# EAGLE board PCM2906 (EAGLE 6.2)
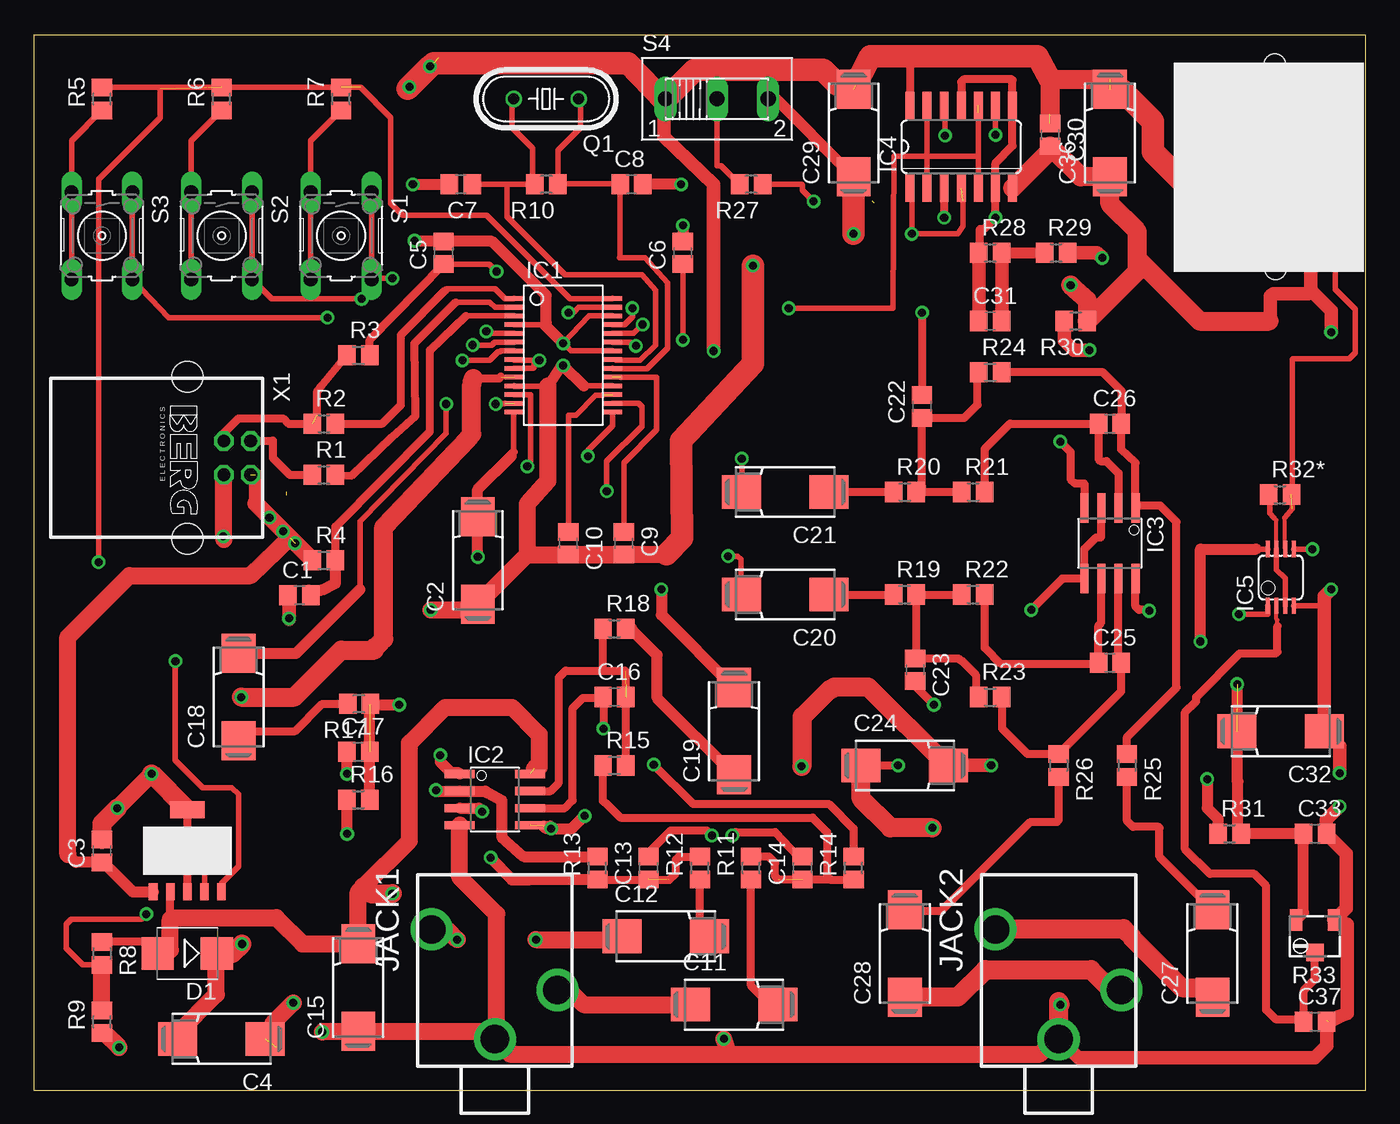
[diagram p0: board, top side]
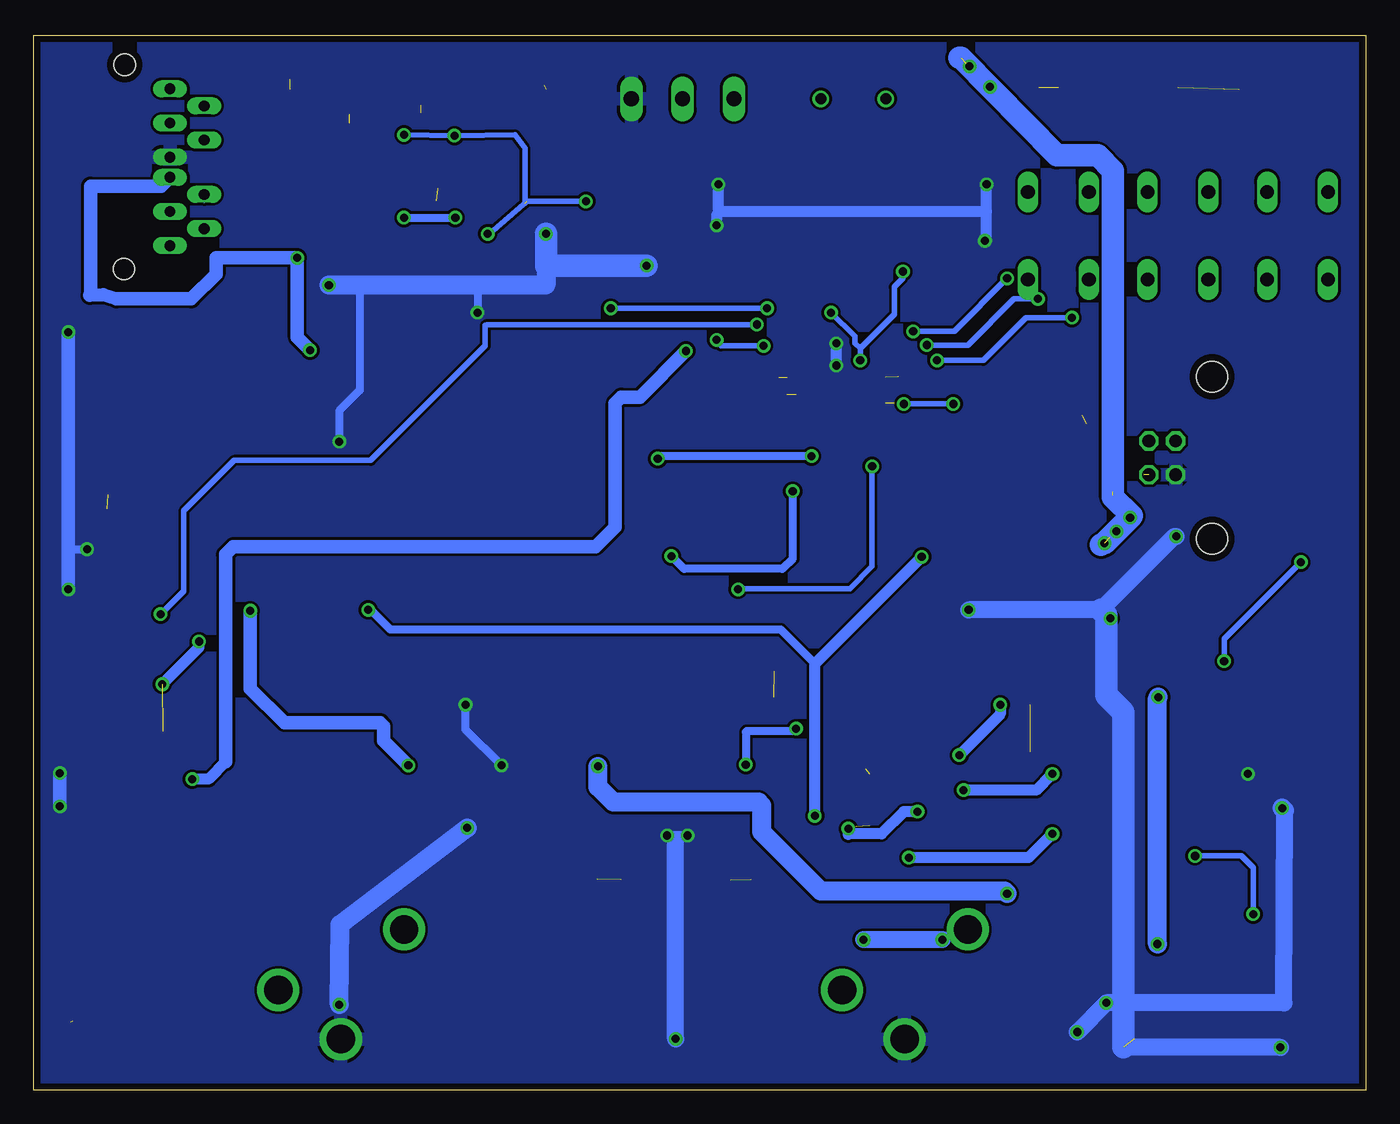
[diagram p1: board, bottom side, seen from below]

Size 99.04 x 78.41 mm. Coordinates in mm from the lower left corner, seen from the top.
Outline: 0,0 99.04,0 99.04,78.41 0,78.41 0,0
Copper layers (1*16): Top 0.035mm / dielectric 1.5mm / Bottom 0.035mm
Design rules: minimum track width 8mil, minimum drill 0.6mm, track to track 8mil, track to pad 8mil, pad to pad 8mil, via to via 8mil, smd to smd 0mil, copper to edge 20mil, drill to drill 10mil, minimum pad ring 8mil, minimum via ring 8mil, stop-mask expansion 0mil, vias tented up to drill 0mil, thermal gap 10mil
Holes 1.6 mm at 92.33,61.02 92.27,76.2

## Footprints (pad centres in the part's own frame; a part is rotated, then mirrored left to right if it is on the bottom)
C2012 = smd 1.3 x 1.5: 1 -0.85,0; 2 0.85,0
085CS_1AR = smd 2.9 x 2.5: + 3.25,0; - -3.25,0
SMB = smd 2.4 x 2.4: A 2.2,0; C -2.2,0
SSOP28DB = smd 0.348 x 1.397: 1 -4.225,-3.656; 2 -3.575,-3.656; 3 -2.925,-3.656; 4 -2.275,-3.656; 5 -1.625,-3.656; 6 -0.975,-3.656; 7 -0.325,-3.656; 8 0.325,-3.656; 9 0.975,-3.656; 10 1.625,-3.656; 11 2.275,-3.656; 12 2.925,-3.656; 13 3.575,-3.656; 14 4.225,-3.656; 15 4.225,3.656; 16 3.575,3.656; 17 2.925,3.656; 18 2.275,3.656; 19 1.625,3.656; 20 0.975,3.656; 21 0.325,3.656; 22 -0.325,3.656; 23 -0.975,3.656; 24 -1.625,3.656; 25 -2.275,3.656; 26 -2.925,3.656; 27 -3.575,3.656; 28 -4.225,3.656
SO08 = smd 0.61 x 2.21: 1 -1.905,-2.616; 2 -0.635,-2.616; 3 0.635,-2.616; 4 1.905,-2.616; 5 1.905,2.616; 6 0.635,2.616; 7 -0.635,2.616; 8 -1.905,2.616
SO14 = smd 0.66 x 2.032: 1 -3.81,-3.073; 2 -2.54,-3.073; 3 -1.27,-3.073; 4 0,-3.073; 5 1.27,-3.073; 6 2.54,-3.073; 7 3.81,-3.073; 8 3.81,3.073; 9 2.54,3.073; 10 1.27,3.073; 11 0,3.073; 12 -1.27,3.073; 13 -2.54,3.073; 14 -3.81,3.073
MSOP08 = smd 0.3 x 1.2: 1 -0.976,-2.113; 2 -0.326,-2.113; 3 0.324,-2.113; 4 0.974,-2.113; 5 0.974,2.112; 6 0.324,2.112; 7 -0.326,2.112; 8 -0.976,2.112
MJ-352 = drill 2.108: P$1 -3.05,-4.7; P$2 1.45,4.65; P$3 5.1,0
HC49/S = drill 0.813: 1 -2.413,0; 2 2.413,0
R2012 = smd 1.3 x 1.5: 1 -0.85,0; 2 0.85,0
3223W = smd 0.9 x 1.6: 1 -1.4,-1.215; 3 1.4,-1.215 | smd 1.3 x 1.3: 2 0,1.215
B3F-10XX = drill 1.016 long: 1 -3.251,2.261; 2 3.251,2.261; 3 -3.251,-2.261; 4 3.251,-2.261
255SB = drill 1.118 long: 1 -3.81,0; 2 0,0; 3 3.81,0
REG103GA-A = smd 1.27 x 0.635: ADJ -3.048,-1.27; EN -3.048,-2.54; GND -3.048,0; IN -3.048,2.54; OUT -3.048,1.27 | smd 1.27 x 2.54: EP 3.048,0
FC300T = drill 0.8 pad 1.27 long: P$1 0,0.75; P$2 0,-0.75; P$3 0,3.29; P$4 0,-3.29; P$5 0,-5.83; P$6 0,5.83; P$7 -2.54,4.56; P$8 -2.54,-4.56; P$9 -2.54,2.02; P$10 -2.54,-2.02
PN61729 = drill 0.95 octagon: 1 1.25,4.71; 2 -1.25,4.71; 3 -1.25,2.71; 4 1.25,2.71 | hole 2.3: -6.02,0; 6.02,0

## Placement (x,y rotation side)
C1  1u  [C2012]  19.75,36.77 0 top
C2  10u  [085CS_1AR]  33.02,39.37 90 top
C3  1u  [C2012]  5.08,17.78 90 top
C4  10u  [085CS_1AR]  13.97,3.81 180 top
C5  1u  [C2012]  30.48,62.23 90 top
C6  1u  [C2012]  48.26,62.23 90 top
C7  30p  [C2012]  31.75,67.31 180 top
C8  30p  [C2012]  44.45,67.31 0 top
C9  1u  [C2012]  43.88,40.64 270 top
C10  1u  [C2012]  39.75,40.64 270 top
C11  10u  [085CS_1AR]  52.07,6.35 0 top
C12  10u  [085CS_1AR]  46.99,11.43 0 top
C13  0.0018u  [C2012]  45.72,16.51 90 top
C14  0.0018u  [C2012]  57.15,16.51 90 top
C15  10u  [085CS_1AR]  24.13,7.62 90 top
C16  330p  [C2012]  43.18,29.21 0 top
C17  330p  [C2012]  24.13,25.15 0 top
C18  10u  [085CS_1AR]  15.24,29.21 90 top
C19  10u  [085CS_1AR]  52.07,26.67 90 top
C20  10u  [085CS_1AR]  55.88,36.83 180 top
C21  10u  [085CS_1AR]  55.88,44.45 180 top
C22  0.0018u  [C2012]  66.04,50.8 90 top
C23  0.0018u  [C2012]  65.53,31.24 270 top
C24  10u  [085CS_1AR]  64.77,24.13 0 top
C25  330p  [C2012]  80.01,31.75 0 top
C26  330p  [C2012]  80.01,49.53 0 top
C27  10u  [085CS_1AR]  87.63,10.16 90 top
C28  10u  [085CS_1AR]  64.77,10.16 90 top
C29  10u  [085CS_1AR]  60.96,71.12 90 top
C30  0.1u  [C2012]  75.56,70.99 270 top
C31  75p  [C2012]  71.12,57.15 0 top
C32  10u  [085CS_1AR]  92.71,26.67 180 top
C33  0.1u  [C2012]  95.25,19.05 0 top
C36  10u  [085CS_1AR]  80.01,71.12 90 top
C37  0.1u  [C2012]  95.25,5.08 0 top
D1  [SMB]  11.43,10.16 180 top
IC1  PCM2906DB  [SSOP28DB]  39.37,54.61 270 top
IC2  OPA2340U  [SO08]  34.29,21.59 270 top
IC3  OPA2340U  [SO08]  80.01,40.64 180 top
IC4  74ACT00D  [SO14]  68.96,70.1 0 top
IC5  OPA2380AIDGKT  [MSOP08]  92.71,38.1 0 top
JACK1  MJ-352WO  [MJ-352]  34.29,8.89 270 top
JACK2  MJ-352WO  [MJ-352]  76.2,8.89 270 top
Q1  12MHz  [HC49/S]  38.1,73.66 180 top
R1  22  [R2012]  21.59,45.72 0 top
R2  22  [R2012]  21.59,49.53 0 top
R3  1.5K  [R2012]  24.13,54.61 0 top
R4  2.2  [R2012]  21.59,39.37 0 top
R5  1.5K  [R2012]  5.08,73.66 90 top
R6  1.5K  [R2012]  13.97,73.66 90 top
R7  1.5K  [R2012]  22.86,73.66 90 top
R8  27K  [R2012]  5.08,10.16 270 top
R9  13K  [R2012]  5.08,5.08 90 top
R10  1M  [R2012]  38.1,67.31 180 top
R11  12K  [R2012]  53.34,16.51 90 top
R12  12K  [R2012]  49.53,16.51 90 top
R13  3.9K  [R2012]  41.91,16.51 90 top
R14  3.9K  [R2012]  60.96,16.51 90 top
R15  12K  [R2012]  43.18,24.13 0 top
R16  12K  [R2012]  24.13,21.59 0 top
R17  100  [R2012]  24.19,28.7 180 top
R18  100  [R2012]  43.18,34.29 0 top
R19  12K  [R2012]  64.77,36.83 0 top
R20  12K  [R2012]  64.77,44.45 0 top
R21  3.9K  [R2012]  69.85,44.45 0 top
R22  3.9K  [R2012]  69.85,36.83 0 top
R23  12K  [R2012]  71.12,29.21 0 top
R24  12K  [R2012]  71.12,53.34 0 top
R25  100  [R2012]  81.28,24.13 270 top
R26  100  [R2012]  76.2,24.13 270 top
R27  1.5K  [R2012]  53.34,67.31 180 top
R28  33  [R2012]  71.12,62.23 0 top
R29  33  [R2012]  76.01,62.23 0 top
R30  270  [R2012]  77.47,57.15 180 top
R31  2.2  [R2012]  88.9,19.05 0 top
R32*  1M  [R2012]  92.65,44.26 0 top
R33  10K  [3223W]  95.25,11.43 180 top
S1  [B3F-10XX]  22.86,63.5 270 top
S2  [B3F-10XX]  13.97,63.5 270 top
S3  [B3F-10XX]  5.08,63.5 270 top
S4  [255SB]  50.8,73.66 0 top
U$1  REG103GA-A  [REG103GA-A]  11.43,17.78 90 top
U$2  FC300T  [FC300T]  88.9,68.58 0 top
X1  [PN61729]  11.43,46.99 270 top

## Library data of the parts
C1-C33 C36 C37 R1-R31 R32* = rcl
D1 = diode
IC1 = texas
IC2 IC3 = burr-brown
IC4 = 74xx-eu
IC5 = linear
JACK1 JACK2 = my_lib
Q1 = crystal
R33 = pot
S1-S3 = switch-omron
S4 = switch
U$1 = My-custom
U$2 = Firecomms
X1 = con-berg

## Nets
GND: C2.- C3.2 C4.- C5.2 C6.2 C7.2 C8.2 C9.2 C10.2 C13.2 C14.2 C15.- C22.2 C23.2 C24.- C29.- C30.2 C32.- C33.2 C36.- IC1.4 IC1.11 IC1.18 IC1.22 IC1.26 IC2.4 IC3.4 IC4.7 IC5.4 IC5.5 JACK1.P$3 JACK2.P$3 R9.1 R30.1 R33.1 S4.3 U$1.EP U$1.GND U$2.P$1 X1.4
N$1: IC1.1 R2.2
N$2: IC1.2 R1.2
N$3: R1.1 X1.2
N$4: R2.1 R3.1 X1.3
N$5: C5.1 IC1.8 IC1.9 IC1.27 R3.2
N$7: IC1.3 R4.2
N$8: C17.2 IC2.1 R16.2 R17.1
N$9: IC1.5 S1.1 S1.2
N$10: R7.1 S1.3 S1.4
N$11: IC1.6 S2.1 S2.2
N$12: IC1.7 S3.1 S3.2
N$13: IC1.28 R5.2 R6.2 R7.2 U$1.EN
N$14: R5.1 S3.3 S3.4
N$15: R6.1 S2.3 S2.4
N$16: C17.1 IC2.2 R13.2
N$17: R8.2 R9.2 U$1.ADJ
N$18: C4.+ D1.C IC1.10
N$19: C6.1 IC1.23
N$20: C7.1 Q1.2 R10.2
N$21: C8.1 IC1.20 Q1.1 R10.1
N$22: C11.+ R11.1
N$23: C9.1 IC1.19
N$24: C11.- JACK1.P$2
N$25: C10.1 IC1.17
N$26: C12.- JACK1.P$1
N$27: C12.+ R12.1
N$28: C13.1 R12.2 R13.1 R16.1
N$29: C15.+ C24.+ D1.A IC2.8 IC3.8 R8.1 U$1.OUT
N$30: C14.1 R11.2 R14.1 R15.1
N$31: C16.1 IC2.6 R14.2
N$32: C20.- R19.1
N$33: C21.- R20.1
N$34: C16.2 IC2.7 R15.2 R18.1
N$35: C28.+ R26.2
N$36: C27.+ R25.2
N$37: C21.+ IC1.15
N$38: C20.+ IC1.16
N$39: C18.- R17.2
N$40: C18.+ IC1.13
N$41: C19.- R18.2
N$42: C19.+ IC1.12
N$43: C31.1 IC4.3 IC4.6 IC4.8 IC4.11 R28.1
N$44: C27.- JACK2.P$1
N$45: C28.- JACK2.P$2
N$46: IC4.1 IC4.4 IC4.9 IC4.12 R27.1
N$47: C22.1 R20.2 R21.1 R24.1
N$48: C23.1 R19.2 R22.1 R23.1
N$49: C31.2 R28.2 R29.1
N$50: C26.1 IC3.2 R21.2
N$51: C25.1 IC3.6 R22.2
N$52: C2.+ IC1.14 IC2.3 IC2.5 IC3.3 IC3.5
N$53: C26.2 IC3.1 R24.2 R25.1
N$54: C25.2 IC3.7 R23.2 R26.1
N$55: R29.2 R30.2 U$2.P$2
N$56: IC1.25 IC4.2 IC4.5 IC4.10 IC4.13
N$57: R27.2 S4.2
N$59: IC5.6 R32*.2 U$2.P$9
N$60: C32.+ C33.1 IC5.8 R31.2 R33.3
N$61: IC1.24 IC5.1
N$67: IC5.2 R33.2
S$2: C3.1 C29.+ C30.1 C36.+ IC4.14 R4.1 R31.1 U$1.IN U$2.P$10 X1.1
S$6: IC5.3 IC5.7

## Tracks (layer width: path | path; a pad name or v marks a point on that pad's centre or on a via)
GND  (via drill 0.6)  (2 unrouted)
  Top 0.254: U$2.P$1 88.9,69.85
  Top 0.406: IC1.26 41.28,57.53 v39.37,55.5 39.93,54.94 IC1.22 | 37.98,56.88 IC1.4 | 40.88,52.34 IC1.18 | IC1.11 35.73,52.32 38.23,52.32 | 39.24,53.85 v39.37,53.85 | 95.04,40.21 IC5.5 | IC5.4 95.85,35.99 95.96,35.88
  Top 0.61: C13.2 45.72,17.65 47.37,19.3 50.04,19.3 v50.42,18.92 | C14.2 56.81,17.36 55.12,19.18 52.2,19.18 v51.94,18.92 | U$1.EP U$1.GND | IC3.4 78.11,45.09 77.41,45.09 77.09,45.4 77.09,47.43 v76.33,48.2 | v66.04,57.78 C22.2 | C23.2 65.53,30.04 v66.93,28.64 | C24.- v64.26,24.13 | v95.06,40.2 95.04,40.21 | 95.96,35.88 95.85,34.59
  Top 0.813: v28.19,67.31 C7.2 | v28.32,63.12 28.36,63.08 C5.2 34.08,63.08 38.1,59.05 38.1,57 37.98,56.88 v39.37,55.5 | v39.37,53.85 40.88,52.34 | 38.23,52.32 39.24,53.85 | v48.13,67.31 C8.2 | v48.26,64.26 C6.2 | S4.3 55.18,73.66 60.58,68.26 60.58,68.25 C29.-
  Top 1.016: U$2.P$1 94.82,69.33 94.93,69.22 94.93,59.44 | 94.93,59.44 94.74,59.18 92.2,59.18 91.95,58.99 91.95,57.24 91.86,57.15 | R33.1 96.72,12.64 96.77,12.7 | 96.77,12.7 97.6,13.53 97.6,17.55 C33.2 96.1,20.09 v97.09,21.08 | v97.09,23.56 97.09,25.54 C32.- 95.96,35.88 95.96,36.72 v96.46,37.21 | v96.46,56.33 96.46,57.91 94.93,59.44 | 96.77,12.7 97.66,12.32 97.66,5.71 97.03,5.46 96.27,5.08 | 96.14,5.14 96.14,3.3 95.25,2.41 77.66,2.41 76.33,3.75
  Top 1.27: 36.69,39.79 C9.2 C10.2 44.47,39.81 47.05,39.81 | 36.69,39.79 C2.- 32.59,35.69 v29.53,35.69 | X1.4 14.14,40.94 v14.1,41.15 | v6.35,3.17 5.29,4.23 R9.1 | JACK2.P$3 75.93,3.79 74.8,2.67 51.69,2.67 | IC2.4 31.67,15.82 34.42,13.08 34.42,4.7 33.9,4.18 | 51.69,2.67 v51.31,3.81 | 51.69,2.67 35.41,2.67 JACK1.P$3 33.9,4.18 | 33.9,4.18 33.71,4.37 C15.- 21.52,4.37 v21.46,4.32 | v6.22,20.95 v8.76,23.5 | v19.3,6.48 17.78,4.95 | 38.23,52.32 38.23,45.28 36.7,43.56 36.7,39.8 36.69,39.79
  Top 1.422: v8.76,23.5 U$1.EP | C3.2 5.08,19.81 v6.22,20.95 | 82.04,61.78 82.04,63.82 80.01,65.85 C36.- 77.84,67.87 C30.2 75.56,69.83 IC4.7 | 82.04,61.78 86.68,57.15 91.86,57.15 | 82.04,61.78 82.04,60.87 R30.1 78.32,58.71 v77.09,59.82 | C24.- 61.52,21.66 63.69,19.49 v66.8,19.49 | v76.33,6.35 76.2,6.6 JACK2.P$3
  Top 1.676: v60.96,63.63 C29.- | v53.47,61.28 53.47,53.98 48.13,48.26 48.2,41.02 47.05,39.81
  Bottom 0.61: v50.42,18.92 v51.94,18.92 | v76.33,48.2 76.33,50.48 74.8,52.01 74.8,59.5 74.49,59.82 | v66.04,57.78 66.04,59.44 66.42,59.82 | v66.93,28.64 66.93,26.8 v64.26,24.13 | 96.46,40.2 v95.06,40.2
  Bottom 0.813: 28.19,65.28 28.19,63.12 v28.32,63.12 | 28.19,65.28 v28.19,67.31 | v39.37,53.85 v39.37,55.5 | v48.13,67.31 48.13,65.28 48.01,65.28 | 28.19,65.28 48.01,65.28 | v48.26,64.26 48.26,65.02 48.01,65.28
  Bottom 1.016: v97.09,23.56 v97.09,21.08 | v96.46,56.33 96.46,40.2 v96.46,37.21
  Bottom 1.27: v14.1,41.15 14.22,41.15 19.68,35.69 v29.53,35.69 | v6.35,3.17 18.03,3.17 | v51.31,3.81 51.31,18.54 | v21.46,4.32 v19.3,6.48 6.1,6.48 6.03,20.77
  Bottom 1.422: 6.03,20.77 v6.22,20.95 | v77.09,59.82 74.49,59.82 66.42,59.82 60.96,59.82 60.96,61.28 | v66.8,19.49 76.26,12.32 v76.33,6.35
  Bottom 1.676: 19.68,35.69 19.3,35.31 19.3,29.34 18.03,28.07 18.03,3.17 | v60.96,63.63 60.96,61.28 v53.47,61.28
  pour Bottom: -0.7,79.31 100.52,79.31 100.52,77.72 100.2,77.72 100.2,-1.84 -1.65,-1.84 -1.65,-0.95 -0.7,-0.95
N$1
  Top 0.406: 30.61,59.44 30.48,59.44 30.73,59.56 34.29,59.56 35.05,58.8 35.68,58.8 IC1.1
  Top 0.61: R2.2 25.91,49.53 27.3,50.93 27.3,56.13 30.61,59.44
N$2
  Top 0.406: 31.37,58.55 33.91,58.55 34.29,58.17 35.7,58.17 IC1.2
  Top 0.61: R1.2 23.62,45.66 26.61,48.51 28.38,50.1 28.32,55.5 31.37,58.55
N$3
  Top 0.254: R1.1 20.32,45.72
  Top 0.61: X1.2 17.76,48.24 17.78,48.26 17.78,46.99 19.05,45.72 R1.1
N$4  (1 unrouted)
  Top 0.61: R3.1 21.38,52.32 21.25,52.11 21.08,51.94 21.08,50.16 | X1.3 14.14,48.81 15.24,49.91 18.54,49.91 18.92,49.53 R2.1
N$5  (via drill 0.6)
  Top 0.406: C5.1 33.87,61.38 v34.42,60.83 | v37.59,54.23 37.08,54.23 | 37.08,54.23 35.77,54.23 IC1.8 | IC1.9 37.12,53.63 37.21,53.72 37.21,54.1 37.08,54.23 | v39.75,57.78 40.13,57.78 40.51,58.17 43.01,58.17 IC1.27
  Top 0.61: R3.2 24.98,55.75 C5.1
  Bottom 0.406: v34.42,60.83 34.42,60.33 35.05,59.69 35.05,57.66 37.59,55.12 | 37.59,55.12 v37.59,54.23 | 37.59,55.12 37.97,55.5 37.97,56.01 v39.75,57.78
N$7
  Top 0.406: 32.13,57.53 IC1.3
  Top 0.61: R4.2 22.44,41.87 29.46,48.96 29.46,54.99 32.13,57.53
  Top 0.813: 22.44,37.81 R4.2
N$8  (via drill 0.6)  (1 unrouted)
  Top 0.813: R16.2 24.98,28.64 | 24.98,28.64 R17.1 | 24.98,28.64 v27.18,28.64 | v30.23,24.89 30.23,24.38 30.99,23.62 31.55,23.62 IC2.1
  Bottom 0.813: v27.18,28.64 27.18,27.94 v30.23,24.89
N$9  (via drill 0.6)
  Top 0.406: IC1.5 34.06,56.23 v33.66,56.39 | v26.67,60.33 25.2,60.33 S1.2 S1.1
  Bottom 0.406: v33.66,56.39 30.61,56.39 v26.67,60.33
N$10
  Top 0.406: S1.4 S1.3 20.6,70.55 R7.1
N$11  (via drill 0.6)
  Top 0.406: IC1.6 34.25,55.59 34.04,55.37 v32.64,55.37 | v24.38,58.8 17.68,58.8 S2.2 S2.1
  Bottom 0.406: v32.64,55.37 29.59,55.37 26.16,58.8 v24.38,58.8
N$12  (via drill 0.6)
  Top 0.406: IC1.7 34.74,54.94 34.67,54.86 34.54,54.86 33.91,54.23 v31.88,54.23 | v21.84,57.4 10.06,57.4 S3.2 S3.1
  Bottom 0.406: v31.88,54.23 28.45,54.23 25.27,57.4 v21.84,57.4
N$13  (via drill 0.6)  (2 unrouted)
  Top 0.406: 9.27,74.51 R5.2 | 9.27,74.51 24.3,74.51 26.54,72.26 26.54,65.91 27.43,65.02 33.66,65.02 39.88,58.8 42.99,58.8 IC1.28 | U$1.EN 13.97,15.37 15.24,16.64 15.24,21.97 14.73,22.48 12.57,22.48 10.54,24.51 v10.54,31.88 | v4.83,39.24 4.83,67.69 9.4,72.26 9.4,74.38 9.27,74.51
  Bottom 0.406: v10.54,31.88 10.54,33.53 v4.83,39.24
N$14
  Top 0.406: S3.4 S3.3 2.82,70.55 R5.1
N$15
  Top 0.406: S2.4 S2.3 11.71,70.55 R6.1
N$16  (via drill 0.6)
  Top 0.813: R13.2 36.42,17.36 34.8,18.8 34.8,21.53 33.78,22.1 33.72,22.1 33.59,22.23 IC2.2 29.97,22.23 v29.91,22.29 | v23.3,23.5 23.3,25.12 C17.1
  Bottom 0.813: v29.91,22.29 24.51,22.29 v23.3,23.5
N$17  (via drill 0.6)
  Top 0.254: U$1.ADJ 12.7,15.24
  Top 0.406: R8.2 3.64,9.31 2.41,10.54 2.41,12.32 2.79,12.7 8,12.7 v8.38,13.08 | v12.7,17.4 U$1.ADJ
  Top 1.27: R9.2 R8.2
  Bottom 0.406: v12.7,17.4 9.27,17.4 8.38,16.51 v8.38,13.08
N$18  (via drill 0.6)  (1 unrouted)
  Top 0.61: 32.7,52.9 34.61,52.9 34.73,53.02
  Top 1.27: C4.+ 10.72,4.24 13.59,7.11 13.59,10.12 D1.C
  Top 1.422: D1.C 14.8,10.16 v15.49,10.86 | v15.43,29.21 19.37,29.21 22.86,32.7 25.34,32.7 25.34,32.89 25.65,33.15 26.04,33.53 26.04,41.85 32.32,48.45 32.58,48.77 32.58,52.45 32.7,52.9
  Bottom 1.422: v15.49,10.86 15.49,29.15 v15.43,29.21
N$19  (via drill 0.6)
  Top 0.406: v48.26,55.75 C6.1 | v44.77,55.31 44.45,55.37 44.39,55.56 43.17,55.56 IC1.23
  Bottom 0.406: v48.26,55.75 48.26,55.63 47.94,55.31 v44.77,55.31
N$20
  Top 0.254: 35.56,73.66 Q1.2
  Top 0.406: 35.56,73.66 35.56,71.5 37.08,69.98 37.08,67.48 R10.2 C7.1
N$21
  Top 0.254: 40.64,73.66 Q1.1
  Top 0.406: 40.64,73.66 40.64,71.5 38.99,69.85 38.99,67.35 | 38.99,67.35 R10.1 | 38.99,67.35 43.56,67.35 C8.1 43.6,61.89 43.56,61.85 45.47,61.85 47.12,60.01 47.12,55.12 45.59,53.59 43.07,53.59 IC1.20
N$22
  Top 0.254: C11.+ 54.74,6.35 54.61,6.35
  Top 0.61: R11.1 53.34,7.75 54.74,6.35
N$23  (1 unrouted)
  Top 0.406: C9.1 43.88,46.61 46.29,49.09 46.29,52.96 43.62,52.96
N$24
  Top 1.27: JACK1.P$2 39.8,7.44 40.89,6.35 C11.-
N$25  (1 unrouted)
  Top 0.406: C10.1 39.75,50.16 40.32,50.16 41.78,51.63 42.29,51.63 42.35,51.69
N$26  (via drill 0.6)
  Top 1.27: JACK1.P$1 30.73,11.94 v31.5,11.18 | v37.34,11.18 42.93,11.18 43.18,11.43 | 43.18,11.43 42.93,11.43 | 43.18,11.43 C12.-
  Bottom 1.27: v31.5,11.18 v37.34,11.18
N$27
  Top 0.254: C12.+ 49.66,11.43 49.53,11.43
  Top 0.61: R12.1 49.53,11.56 49.66,11.43
N$28  (via drill 0.6)  (1 unrouted)
  Top 0.254: R13.1 41.91,15.24
  Top 0.61: R12.2 47.97,17.36 47.75,17.14 47.75,16.13 47.24,15.62 41.95,15.62 R13.1
  Top 0.813: R13.1 37.81,15.66 36.83,15.62 35.56,15.62 v33.97,17.27 | v23.3,19.05 23.3,21.57 R16.1
  Bottom 0.813: v33.97,17.27 25.08,17.27 v23.3,19.05
N$29  (via drill 0.6)  (1 unrouted)
  Top 0.254: D1.A 9.91,10.16 10.16,10.16 | R8.1 5.08,11.43
  Top 0.61: 10.16,12.7 U$1.OUT | 9.91,10.16 10.16,10.41 | D1.A 8.89,10.16 8.26,11.05 5.12,11.05 R8.1 | IC3.8 81.92,35.94 82.17,35.69 82.87,35.69 v82.93,35.62
  Top 1.016: C24.+ v71.18,24.13
  Top 1.27: 10.16,10.41 10.16,12.7 10.29,12.83 18.03,12.83 19.99,10.87 C15.+ 24.13,14.73 24.51,15.11 27.94,18.54 27.94,25.78 30.61,28.45 35.56,28.45 37.59,26.42 37.59,24 37.34,24 37.21,23.88
  Top 1.422: C24.+ 67.88,24.13 62.04,29.97 59.5,29.97 59.31,29.78 59.18,29.78 57.15,27.75 57.15,24.13 v57.09,24.07 | v26.67,14.61 25.02,14.61 24.51,15.11
  Bottom 1.016: v82.93,35.62 82.93,29.84 80.39,27.3 73.28,27.3 73.03,27.05 73.03,25.97 v71.18,24.13
  Bottom 1.422: v57.09,24.07 57.09,22.54 55.94,21.4 45.15,21.4 44.9,21.14 44.9,19.18 40.51,14.8 26.86,14.8 v26.67,14.61
N$30  (1 unrouted)
  Top 0.61: R11.2 54.65,17.36 55.12,16.89 55.12,15.88 55.37,15.62 59.31,15.62 | 59.31,15.62 60.92,15.62 R14.1 | R15.1 42.33,21.49 42.48,21.34 42.55,21.34 43.62,20.26 57.91,20.26 58.99,19.18 58.99,15.94 59.31,15.62
N$31  (via drill 0.6)
  Top 0.254: C16.1 41.91,29.21
  Top 0.61: IC2.6 39.5,20.95 40.07,21.53 40.07,28.38 40.83,29.15 42.27,29.15 C16.1 42.35,29.19 v42.35,26.86 | R14.2 60.96,19.43 59.12,21.27 49.02,21.27 v46.1,24.19
  Bottom 0.61: v46.1,24.19 46.1,26.61 46.04,26.67 42.55,26.67 v42.35,26.86
N$32
  Top 0.61: C20.- R19.1
N$33
  Top 0.61: C21.- R20.1
N$34  (1 unrouted)
  Top 0.254: R15.2 44.45,24.13 | R18.1 41.91,34.29 | C16.2 44.45,29.21
  Top 0.61: IC2.7 38.42,22.23 39.05,22.86 39.05,30.67 39.56,31.18 42.42,31.18 | 42.42,31.18 43.94,31.18 44.01,31.11 44.01,24.15 R15.2 | R18.1 42.33,31.27 42.42,31.18
N$35
  Top 0.61: R26.2 76.2,20.07 76.07,19.94 74.11,19.94 67.5,13.34 64.84,13.34 C28.+
N$36
  Top 0.61: R25.2 81.28,20 81.72,19.56 83.63,19.56 83.69,19.49 83.69,17.35 C27.+
N$37  (via drill 0.6)
  Top 0.406: IC1.15 43.03,49.38 41.21,47.56 v41.21,47.12 | v52.64,46.93 52.64,44.46 C21.+
  Bottom 0.406: 52.45,47.12 v52.64,46.93
  Bottom 0.61: v41.21,47.12 52.45,47.12
N$38  (via drill 0.6)
  Top 0.406: IC1.16 44.98,51.03 45.21,50.8 45.21,49.34 42.61,46.74 v42.61,44.51 | v51.63,39.69 52.32,39.69 52.58,39.43 52.58,36.88 C20.+
  Bottom 0.61: v42.61,44.51 42.61,39.5 43.37,38.73 50.67,38.73 v51.63,39.69
N$39
  Top 0.254: C18.- 15.24,26.67
  Top 0.61: 15.24,26.67 19.43,26.67 21.46,28.7 R17.2
N$40  (via drill 0.6)  (1 unrouted)
  Top 0.406: 24.26,37.21 24.26,42.29 30.67,48.83 v30.67,50.99 | v34.35,50.99 34.99,50.99 35.05,51.05
  Top 0.813: C18.+ 19.51,32.46 24.26,37.21
  Bottom 0.406: v30.67,50.99 v34.35,50.99
N$41
  Top 0.254: 44.45,34.29 R18.2
  Top 0.813: 44.45,34.29 44.45,34.23 46.35,32.32 46.35,29.14 C19.-
N$42  (via drill 0.6)
  Top 0.406: IC1.12 36.89,51.69 36.96,51.69 36.96,46.67 v36.7,46.35
  Top 0.813: v46.67,37.21 46.67,35.32 C19.+
  Bottom 0.406: v36.7,46.35 36.7,38.92 38.35,37.27 46.61,37.27 v46.67,37.21
N$43  (via drill 0.6)
  Top 0.254: C31.1 69.85,57.15 | R28.1 69.85,62.23
  Top 0.61: IC4.11 68.96,74.93 69.15,75.12 72.71,75.12 72.77,75.06 IC4.8 72.77,70.17 71.5,68.9 IC4.6 v71.5,64.83 70.67,64.01 70.36,64.01 70.36,62.23 R28.1 | v67.69,64.83 IC4.3
  Top 1.016: C31.1 R28.1
  Bottom 0.61: v71.5,64.83 v67.69,64.83
N$44
  Top 0.254: 87.63,7.62 C27.-
  Top 1.422: 87.63,7.62 85.34,7.62 81.66,11.3 81.66,11.37 81.03,12 71.56,12 JACK2.P$1
N$45
  Top 1.422: JACK2.P$2 80.13,7.44 78.61,8.95 70.74,8.95 68.71,6.92 64.78,6.92 C28.-
N$46  (via drill 0.6)  (2 unrouted)
  Top 0.406: R27.1 57.09,67.31 57.15,67.25 57.15,66.86 v57.98,66.04 | 69.09,66.1 69.09,64.2 68.71,63.63 v65.28,63.63 65.28,67.03 IC4.1 | IC4.12 67.75,73.18 v67.75,70.93 | v71.5,70.99 IC4.9
  Bottom 0.406: v57.98,66.04 62.36,66.04 65.15,63.63 v65.28,63.63 | 62.51,65.9 62.51,69.98 63.25,70.99 v67.75,70.93 v71.5,70.99
N$47
  Top 0.254: R21.1 68.58,44.45
  Top 0.61: R21.1 R20.2 66.04,44.87 C22.1 69.19,49.95 70.17,50.93 70.17,53.24 R24.1
N$48
  Top 0.61: R22.1 R19.2 65.62,32.18 C23.1 68.75,32.09 68.9,31.94 68.96,31.94 70.04,30.86 70.04,29.44 R23.1
N$49
  Top 0.813: R28.2 R29.1
  Top 1.016: C31.2 R28.2
N$50
  Top 0.61: R21.2 70.7,47.65 72.58,49.53 C26.1 79.16,46.89 79.31,46.74 79.76,46.74 80.64,45.85 IC3.2
N$51
  Top 0.254: C25.1 78.74,31.75
  Top 0.61: R22.2 70.7,32.87 71.88,31.69 79.1,31.69 C25.1 79.16,34.52 79.38,34.73 IC3.6
N$52  (via drill 0.6)  (1 unrouted)
  Top 0.406: 35.69,47.43 35.69,50.36 IC1.14
  Top 0.61: 35.5,47.12 35.5,47.24 35.69,47.43 | IC3.3 79.38,41.15 79.31,41.08 78.99,41.08 78.11,40.2 IC3.5 76.47,38.02 76.47,37.99 v74.17,35.69
  Top 0.813: 35.5,47.12 33.02,44.64 C2.+ v33.02,39.62 | IC2.3 33.08,20.95 v33.34,20.7 | v38.48,19.43 38.1,19.43 37.91,19.62 38.42,19.62 38.61,19.43 40.01,19.43 v40.96,20.38
  Bottom 0.61: v74.17,35.69 73.98,35.69 72.52,34.23 43.5,34.23 40.96,31.69
  Bottom 0.813: v33.34,20.7 34.35,20.7 36.01,19.05 38.42,19.05 38.48,18.99 v38.48,19.43 | v40.96,20.38 40.96,31.69 v33.02,39.62
N$53
  Top 0.61: R24.2 79.5,53.34 80.9,51.94 80.9,49.57 C26.2 80.86,47.6 81.92,46.61 IC3.1 82.09,43.43 83.76,43.43 84.96,42.23 84.96,29.91 81.28,26.23 R25.1
N$54
  Top 0.61: IC3.7 80.64,31.96 C25.2 80.86,29.64 R26.1 73.89,24.98 72.01,26.86 72.01,29.17 R23.2
N$55  (via drill 0.6)
  Top 1.016: R29.2 79.06,62.23 v79.44,61.85 | v78.49,54.99 77.34,54.99 76.64,55.69 76.64,57.13 R30.2
  Bottom 1.016: v78.49,54.99 79.44,55.94 v79.44,61.85 85.47,61.85 85.47,60.64 87.31,58.8 92.9,58.8 93.85,59.12 94.87,59.05 94.81,59.12 94.81,67.18 89.55,67.18 U$2.P$2
N$56  (via drill 0.6)  (1 unrouted)
  Top 0.406: IC1.25 43.93,56.88 44.51,57.47 v44.51,58.1 | 70.23,69.41 70.23,72.64 | 70.23,69.41 IC4.5 | 66.42,69.41 70.23,69.41 | 66.42,69.41 IC4.13 | v56.13,58.1 63.88,58.1 63.94,69.41 66.42,69.41 | 66.42,69.41 IC4.2
  Bottom 0.406: v44.51,58.1 v56.13,58.1
N$57
  Top 0.406: S4.2 50.8,68.71 51.09,68.71 R27.2
N$59  (1 unrouted)
  Top 0.254: IC5.6 93.03,40.28
  Top 0.305: 93.03,40.28 93.03,42.55
  Top 0.406: 93.03,42.55 93.56,43.2 93.56,54.29 93.62,54.36 97.79,54.36 98.23,54.8 98.23,58.04 96.77,59.5 96.77,68.96 95.14,70.6 U$2.P$9
N$60  (via drill 0.6)  (1 unrouted)
  Top 0.406: IC5.8 90.89,40.21 90.87,40.2
  Top 0.813: 90.87,40.2 86.74,40.2 v86.74,33.34 | v89.47,30.16 89.47,22.99 89.53,22.92 89.53,19.27 R31.2 C33.1 94.4,13.2 R33.3
  Bottom 0.813: v86.74,33.34 86.74,32.89 v89.47,30.16
N$61  (via drill 0.6)
  Top 0.406: IC1.24 44.61,56.23 v45.28,56.9 | v89.6,35.37 91.76,35.37 91.76,35.96 IC5.1
  Bottom 0.406: v45.28,56.9 65.34,56.9 65.47,56.83 65.47,55.31 73.98,46.8 84.14,46.8 87.88,43.05 87.88,37.08 v89.6,35.37
N$67
  Top 0.305: 92.46,34.48 92.46,34.92 92.39,34.99 92.39,35.98 IC5.2
  Top 0.61: R33.2 95.25,8.26 94.42,7.43 94.42,5.33 94.36,5.27 92.33,5.27 91.63,5.97 91.63,15.18 90.74,16.07 87.44,16.07 85.6,17.91 85.6,28.07 86.42,28.89 86.42,29.21 89.66,32.45 92.33,32.45 92.46,32.58 92.46,34.48
S$1
  Top 0.813: 22.42,37.66 21.4,37.15 20.45,37.15
S$2  (via drill 0.6)  (7 unrouted)
  Top 0.254: R4.1 20.32,39.37
  Top 0.61: 65.15,76.83 IC4.14
  Top 0.813: 2.54,17.53 3.14,16.93 C3.1 5.17,16.93 7.37,14.73 U$1.IN | R31.1 88.05,20.15 87.25,20.95 v87.25,23.11
  Top 1.016: 16.51,43.6 16.51,45.72 | v50.55,54.93 50.55,67.31 46.86,70.87 46.86,73.53
  Top 1.27: 19.07,41.04 R4.1 | 19.07,41.04 16.51,43.6 | 19.07,41.04 16.13,38.23 7.11,38.23 2.54,33.66 2.54,17.53
  Top 1.422: 60.5,74.37 C29.+ | 75.56,72.52 75.56,75.12 80.01,75.12
  Top 1.676: 27.81,74.42 v27.94,74.55 v29.46,76.07 29.72,76.33 44.2,76.33 46.86,73.53 49.15,75.82 58.67,75.82 59.82,74.68 61.09,74.68 | C29.+ 62.22,76.83 65.15,76.83 74.61,76.83 75.56,75.12 | C36.+ 80.82,74.37 83.19,72.01 83.19,69.73 U$2.P$10
  Bottom 0.254: U$2.P$10 86.36,66.04
  Bottom 0.813: v87.25,23.11 86.04,23.11 84.77,24.38
  Bottom 1.016: 84.77,24.38 84.77,39.81 84.2,40.39 57.28,40.39 55.82,41.85 55.82,51.05 55.37,51.5 53.98,51.5 v50.55,54.93
  Bottom 1.676: 30.23,76.71 30.1,76.71 22.99,69.47 19.94,69.47 18.8,68.33 18.8,44.45 | 18.8,44.2 18.8,44.07 17.4,42.67 v19.43,40.64 19.68,40.51
S$3
  Top 0.406: 35.18,67.18 35.18,64.9 39.5,60.58 45.21,60.58 46.23,59.44 46.23,55.37 45.09,54.23 43.31,54.23
S$4  (via drill 0.6)
  Top 1.016: 18.99,36.45 v18.99,35.05 18.99,34.99
S$5
  Top 0.406: 46.86,73.53 46.86,73.66
S$6
  Top 0.305: 92.2,42.55 92.39,42.35 92.39,40.27 IC5.7
  Top 0.406: 91.89,43.62 91.89,42.86 92.2,42.55 | IC5.7 92.39,40.2 92.39,38.67 93.03,38.03 IC5.3
S$8  (via drill 0.6)
  other vias: 18.54,41.53
S$9  (via drill 0.6)
  other vias: 17.53,42.55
